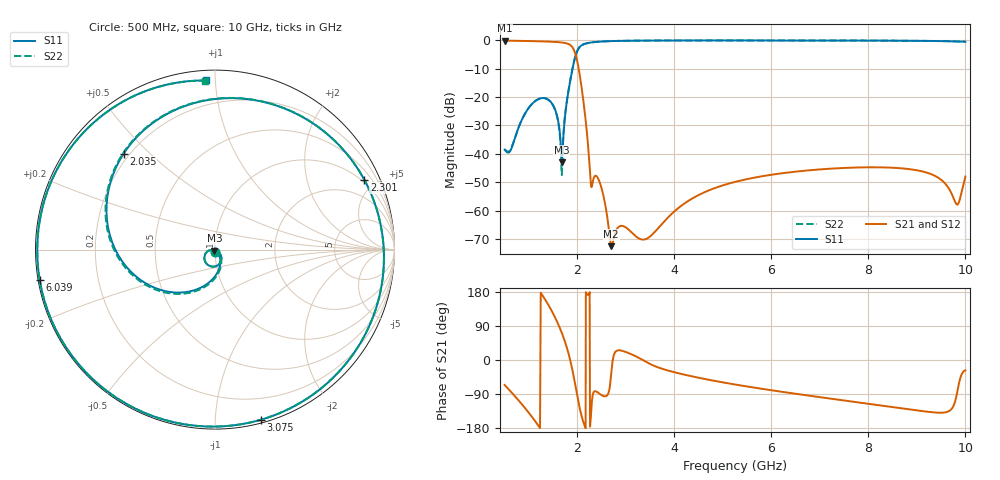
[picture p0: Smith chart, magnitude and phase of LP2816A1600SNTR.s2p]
! Created Mon Mar 25 09:31:35 2019
!	AVX THIN FILM OPERATION
!	LP2816S High Performance Low Pass Filters
!	P/N LP2816A1600SNTR
! Created  10 January 2017
! List of port names and net name(s): example Port n = <port_name> <net_name1> <net_name2> ...
! Port 1 = P1 P1
! Port 2 = P2 P2
# mhz S db R 50
! 2 Port Network Data from data block
! freq  dbS11  angS11  dbS21  angS21  dbS12  angS12  dbS22  angS22
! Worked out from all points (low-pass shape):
!   485 points, 500 MHz to 10 GHz, reference 50 ohm
!   highest |S21| = -0.13 dB at 500 MHz (marker M1); lowest = -72.5 dB at 2.698 GHz (marker M2)
!   |S21| within 3 dB of the highest: start of sweep to 1.921 GHz
!   lowest |S11| = -42.9 dB at 1.68 GHz (marker M3), VSWR 1.01, Z = 49.6 - j0.619 ohm
!   |S11| at or under -10 dB: start of sweep to 1.9 GHz
!   |S22| runs from -47.5 to -0.1 dB; largest |S21 - S12| = 0
!   S11 on the Smith chart (normalised r, x): 500 MHz: 1.00, -0.02; 2.035 GHz: 0.18, +0.42; 2.301 GHz: 0.87, +4.33; 3.075 GHz: 0.02, -1.31; 6.039 GHz: 0.00, -0.09; 10 GHz: 0.05, +0.94
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500  -38.54 -97.0  -0.13 -65.8  -0.13 -65.8  -38.36 -96.2
858.0729  -27.90 -41.1  -0.22 -117.1  -0.22 -117.1  -27.85 -42.3
1216.146  -20.57 -89.2  -0.37 -177.0  -0.37 -177.0  -20.58 -90.2
1548.438  -24.72 -156.0  -0.59 110.1  -0.59 110.1  -24.90 -158.1
1680  -42.91 -119.4  -0.78 71.3  -0.78 71.3  -47.46 -100.3
1740  -27.69 -55.4  -0.93 50.0  -0.93 50.0  -27.34 -50.1
1853.333  -14.19 -102.6  -1.67 -0.8  -1.67 -0.8  -14.06 -100.8
1945  -6.57 -162.2  -4.07 -57.8  -4.07 -57.8  -6.51 -161.0
2035  -2.64 133.7  -10.79 -119.2  -10.79 -119.2  -2.62 134.4
2085  -1.80 104.2  -16.36 -146.9  -16.36 -146.9  -1.79 104.8
2300.625  -0.74 25.1  -51.28 -107.8  -51.28 -107.8  -0.74 25.4
2462.292  -0.47 -8.7  -50.09 -89.5  -50.09 -89.5  -0.48 -8.6
2698.056  -0.28 -41.5  -72.49 -36.0  -72.49 -36.0  -0.29 -41.4
3075.278  -0.16 -74.9  -66.96 17.3  -66.96 17.3  -0.16 -74.8
3695  -0.09 -108.2  -65.60 -20.9  -65.60 -20.9  -0.09 -108.2
5311.667  -0.07 -155.5  -49.60 -66.0  -49.60 -66.0  -0.07 -155.5
6039.167  -0.08 -170.1  -47.25 -80.6  -47.25 -80.6  -0.08 -170.0
6847.5  -0.09 175.4  -45.68 -95.4  -45.68 -95.4  -0.08 175.4
8446.204  -0.13 146.3  -44.84 -123.4  -44.84 -123.4  -0.13 146.3
9389.259  -0.26 121.5  -47.88 -138.7  -47.88 -138.7  -0.26 121.6
9811.389  -0.40 103.9  -57.65 -97.8  -57.65 -97.8  -0.40 104.1
10000  -0.50 93.2  -48.00 -27.1  -48.00 -27.1  -0.51 93.5
